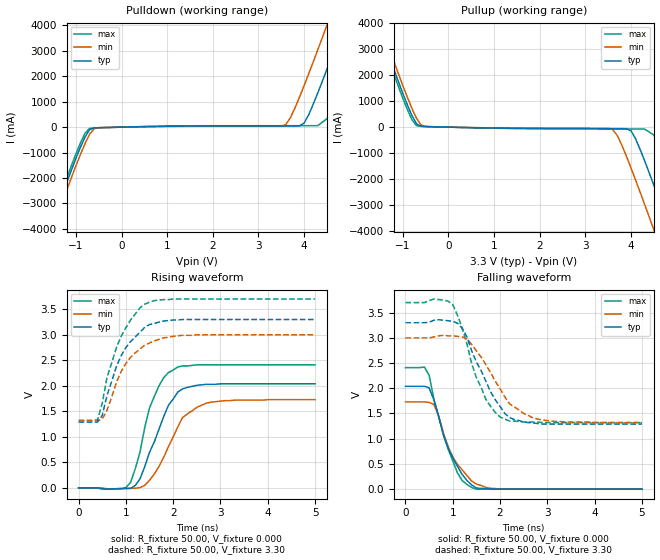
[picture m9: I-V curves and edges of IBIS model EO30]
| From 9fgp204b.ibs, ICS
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|   Model EO30
[Model]   EO30
Model_type   Output
Polarity   Non-Inverting
Vmeas =   1.50V
Cref =  30.00pF
Rref =  83.000
Vref =   1.50V
C_comp   3.40pF   2.85pF   3.95pF
[Temperature Range]   27.00   70.00   0.000
[Voltage Range]   3.30V   3.00V   3.70V
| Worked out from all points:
|   slope of the pulldown table from 0 to 0.495 V, typ, clamps not added: 24.6 ohm
|   slope of the pullup table from 0 to 0.495 V, typ, clamps not added: 25.7 ohm
|   rising waveform, R_fixture 50.00, V_fixture 0.000: 20-80 % time 515ps typ, 555ps min, 435ps max; typ from 0 V to 2.04 V
|   rising waveform, R_fixture 50.00, V_fixture 3.30: 20-80 % time 561ps typ, 568ps min, 529ps max; typ from 1.29 V to 3.3 V
|   falling waveform, R_fixture 50.00, V_fixture 0.000: 20-80 % time 483ps typ, 509ps min, 462ps max; typ from 2.04 V to 0 V
|   falling waveform, R_fixture 50.00, V_fixture 3.30: 20-80 % time 616ps typ, 693ps min, 506ps max; typ from 3.3 V to 1.29 V
[Pulldown]
| voltage   I(typ)   I(min)   I(max)
-3.3V     -12.43A    -12.7A     -12.26A
-1.7V     -4.56A     -4.85A     -4.38A
-1.5V     -3.59A     -3.88A     -3.41A
-900mV    -790mA     -1.07A     -620mA
-700mV    -100mA     -280mA     -48.4mA
3.6V      45.57mA    100mA      56.17mA
4V        160mA      1.63A      56.35mA
4.3V      1.34A      3.04A      57.15mA
4.5V      2.27A      4A         330mA
4.9V      4.19A      5.94A      2.1A
5.3V      6.15A      7.9A       4.02A
6.6V      12.57A     14.32A     10.42A
[Pullup]
| voltage   I(typ)   I(min)   I(max)
-3.3V     12.5A      12.78A     12.33A
-1.7V     4.63A      4.93A      4.45A
-1.5V     3.66A      3.96A      3.48A
-700mV    130mA      340mA      58.94mA
-500mV    22.21mA    22.78mA    24.27mA
3.6V      -57.14mA   -89.68mA   -71.87mA
4V        -140mA     -1.56A     -72.83mA
4.3V      -1.29A     -2.97A     -74.15mA
4.5V      -2.22A     -3.93A     -300mA
4.9V      -4.13A     -5.87A     -2.05A
5.3V      -6.08A     -7.82A     -3.97A
6.6V      -12.49A    -14.23A    -10.36A
[Ramp]
| variable   typ   min   max
dV/dt_r   1.22/0.49n   1.04/0.60n   1.45/0.43n
dV/dt_f   1.21/0.60n   1.01/0.71n   1.43/0.50n
R_load = 50.00
[Rising Waveform]
R_fixture = 50.00
V_fixture = 0.000
V_fixture_min = 0.000
V_fixture_max = 0.000
| time   V(typ)   V(min)   V(max)
0s        0V         0V         0V
900ps     -12.49mV   -13mV      -15mV
1.1ns     -7.67mV    -9.23mV    110mV
1.3ns     180mV      6.48mV     710mV
1.5ns     700mV      150mV      1.57V
1.8ns     1.4V       600mV      2.16V
2.1ns     1.88V      1.2V       2.37V
2.3ns     1.97V      1.45V      2.39V
2.8ns     2.03V      1.68V      2.41V
5ns       2.04V      1.73V      2.41V
[Rising Waveform]
R_fixture = 50.00
V_fixture = 3.30
V_fixture_min = 3.00
V_fixture_max = 3.70
| time   V(typ)   V(min)   V(max)
0s        1.29V      1.32V      1.32V
400ps     1.29V      1.32V      1.33V
500ps     1.42V      1.35V      1.66V
600ps     1.81V      1.52V      2.16V
800ps     2.38V      2.07V      2.75V
1ns       2.75V      2.44V      3.14V
1.4ns     3.15V      2.8V       3.6V
1.6ns     3.22V      2.88V      3.67V
2.2ns     3.3V       2.99V      3.7V
5ns       3.3V       3V         3.7V
[Falling Waveform]
R_fixture = 50.00
V_fixture = 0.000
V_fixture_min = 0.000
V_fixture_max = 0.000
| time   V(typ)   V(min)   V(max)
0s        2.04V      1.73V      2.41V
400ps     2.04V      1.73V      2.42V
500ps     2.01V      1.72V      2.26V
600ps     1.77V      1.68V      1.79V
700ps     1.45V      1.46V      1.44V
900ps     820mV      850mV      800mV
1.1ns     450mV      490mV      320mV
1.4ns     84mV       160mV      32.33mV
1.9ns     1.76mV     10.48mV    1.14mV
5ns       -25.18uV   -13.77uV   9.94uV
[Falling Waveform]
R_fixture = 50.00
V_fixture = 3.30
V_fixture_min = 3.00
V_fixture_max = 3.70
| time   V(typ)   V(min)   V(max)
0s        3.3V       3V         3.7V
600ps     3.35V      3.02V      3.77V
1ns       3.33V      3.04V      3.66V
1.2ns     3.19V      3.02V      3.19V
1.5ns     2.52V      2.74V      2.21V
1.7ns     2.14V      2.47V      1.78V
2ns       1.64V      1.99V      1.43V
2.2ns     1.42V      1.69V      1.35V
2.7ns     1.31V      1.41V      1.33V
5ns       1.29V      1.32V      1.32V
